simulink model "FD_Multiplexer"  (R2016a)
settings: Solver=ode3  StartTime=0.0  StopTime=6  FixedStep=1/5000000  RelTol=1e-3
libraries: commsynccomp2 x4, simulink x4

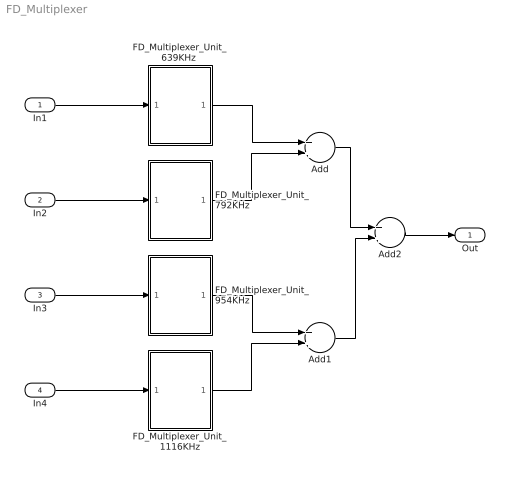
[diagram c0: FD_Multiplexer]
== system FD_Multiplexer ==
  In1 : Inport
  In2 : Inport  Port=2
  In3 : Inport  Port=3
  In4 : Inport  Port=4
  Add : Sum
  Add1 : Sum
  Add2 : Sum
  FD_Multiplexer_Unit_1116KHz : Subsystem
  "FD_Multiplexer_Unit_639KHz " : Subsystem
  FD_Multiplexer_Unit_792KHz : Subsystem
  FD_Multiplexer_Unit_954KHz : Subsystem
  Out : Outport
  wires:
  FD_Multiplexer_Unit_792KHz/1(Output) -> Add/2
  "FD_Multiplexer_Unit_639KHz "/1(Output) -> Add/1
  Add/1 -> Add2/1
  Add2/1 -> Out/1
  In2/1 -> FD_Multiplexer_Unit_792KHz/1(Input)
  In1/1 -> "FD_Multiplexer_Unit_639KHz "/1(Input)
  FD_Multiplexer_Unit_954KHz/1(Output) -> Add1/1
  FD_Multiplexer_Unit_1116KHz/1(Output) -> Add1/2
  In3/1 -> FD_Multiplexer_Unit_954KHz/1(Input)
  In4/1 -> FD_Multiplexer_Unit_1116KHz/1(Input)
  Add1/1 -> Add2/2

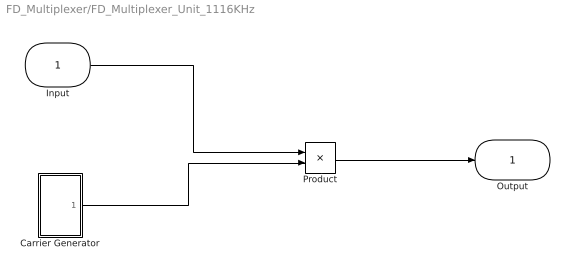
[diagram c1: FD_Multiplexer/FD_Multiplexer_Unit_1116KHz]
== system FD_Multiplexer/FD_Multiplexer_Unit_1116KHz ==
  Input : Inport
  Carrier Generator : Subsystem
  Product : Product
  Output : Outport
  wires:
  Input/1 -> Product/1
  Product/1 -> Output/1
  Carrier Generator/1(Carrier) -> Product/2

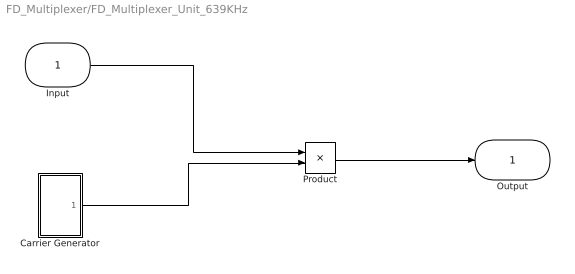
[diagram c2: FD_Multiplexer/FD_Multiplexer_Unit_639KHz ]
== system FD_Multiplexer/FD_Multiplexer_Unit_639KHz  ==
  Input : Inport
  Carrier Generator : Subsystem
  Product : Product
  Output : Outport
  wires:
  Product/1 -> Output/1
  Input/1 -> Product/1
  Carrier Generator/1(Carrier) -> Product/2

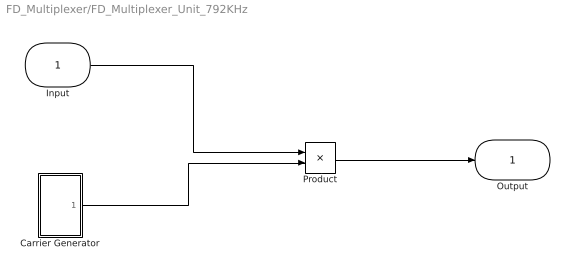
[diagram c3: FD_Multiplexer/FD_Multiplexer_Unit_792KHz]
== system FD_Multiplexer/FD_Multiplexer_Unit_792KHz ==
  Input : Inport
  Carrier Generator : Subsystem
  Product : Product
  Output : Outport
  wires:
  Product/1 -> Output/1
  Input/1 -> Product/1
  Carrier Generator/1(Carrier) -> Product/2

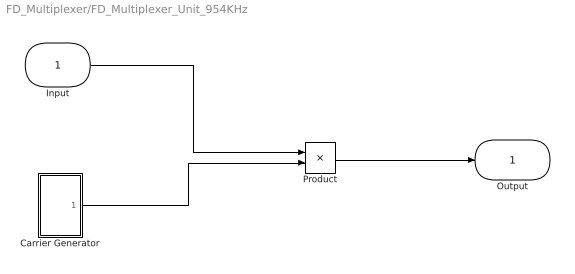
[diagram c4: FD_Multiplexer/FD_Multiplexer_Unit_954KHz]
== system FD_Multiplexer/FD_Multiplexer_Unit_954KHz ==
  Input : Inport
  Carrier Generator : Subsystem
  Product : Product
  Output : Outport
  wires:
  Input/1 -> Product/1
  Product/1 -> Output/1
  Carrier Generator/1(Carrier) -> Product/2

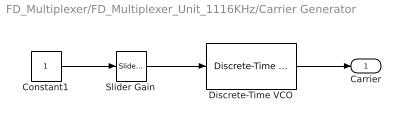
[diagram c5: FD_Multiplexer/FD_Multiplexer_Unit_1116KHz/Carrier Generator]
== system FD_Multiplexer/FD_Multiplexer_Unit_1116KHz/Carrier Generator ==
  Constant1 : Constant
  Discrete-Time VCO : commsynccomp2/Discrete-Time VCO  Ac=1  Fc=0  Kc=1000  Ph=0  ts=1/5000000
  Slider Gain : simulink/Math Operations/Slider Gain  low=550  gain=616  high=2500
  Carrier : Outport
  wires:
  Discrete-Time VCO/1 -> Carrier/1
  Slider Gain/1 -> Discrete-Time VCO/1
  Constant1/1 -> Slider Gain/1

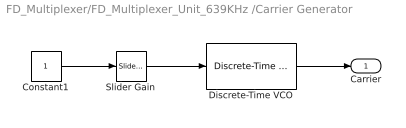
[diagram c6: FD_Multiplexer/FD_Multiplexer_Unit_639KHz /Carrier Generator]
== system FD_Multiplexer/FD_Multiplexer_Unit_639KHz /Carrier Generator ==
  Constant1 : Constant
  Discrete-Time VCO : commsynccomp2/Discrete-Time VCO  Ac=1  Fc=0  Kc=1000  Ph=0  ts=1/5000000
  Slider Gain : simulink/Math Operations/Slider Gain  low=0  gain=139  high=1605
  Carrier : Outport
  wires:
  Discrete-Time VCO/1 -> Carrier/1
  Slider Gain/1 -> Discrete-Time VCO/1
  Constant1/1 -> Slider Gain/1

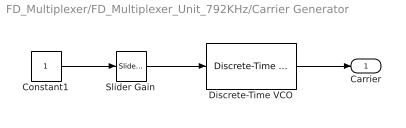
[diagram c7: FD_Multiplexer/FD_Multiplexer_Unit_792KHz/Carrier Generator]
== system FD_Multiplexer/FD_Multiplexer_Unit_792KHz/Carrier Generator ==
  Constant1 : Constant
  Discrete-Time VCO : commsynccomp2/Discrete-Time VCO  Ac=1  Fc=0  Kc=1000  Ph=0  ts=1/5000000
  Slider Gain : simulink/Math Operations/Slider Gain  low=292  gain=292  high=1605
  Carrier : Outport
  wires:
  Discrete-Time VCO/1 -> Carrier/1
  Slider Gain/1 -> Discrete-Time VCO/1
  Constant1/1 -> Slider Gain/1

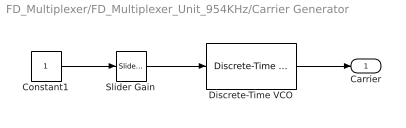
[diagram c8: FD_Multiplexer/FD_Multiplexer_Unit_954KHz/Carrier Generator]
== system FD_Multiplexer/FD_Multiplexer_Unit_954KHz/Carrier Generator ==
  Constant1 : Constant
  Discrete-Time VCO : commsynccomp2/Discrete-Time VCO  Ac=1  Fc=0  Kc=1000  Ph=0  ts=1/5000000
  Slider Gain : simulink/Math Operations/Slider Gain  low=454  gain=454  high=1605
  Carrier : Outport
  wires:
  Discrete-Time VCO/1 -> Carrier/1
  Slider Gain/1 -> Discrete-Time VCO/1
  Constant1/1 -> Slider Gain/1
